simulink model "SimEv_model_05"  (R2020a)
settings: Solver=VariableStepAuto  StartTime=0.0  StopTime=10.0  RelTol=1e-3
undefined symbols (not defined in the file): m, n

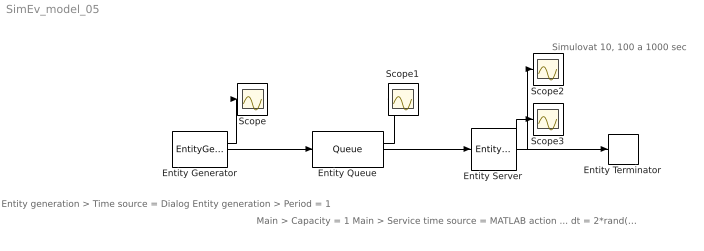
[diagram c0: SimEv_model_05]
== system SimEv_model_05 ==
  note: Simulovat 10, 100 a 1000 sec
  note: Entity generation > Time source = Dialog Entity generation > Period = 1
  note: Main > Capacity = 1 Main > Service time source = MATLAB action ... dt = 2*rand(1,1)
  Entity Generator : EntityGenerator  OutputPortMessageModes=n,m  IntergenerationTimeAction=|  NumberEntitiesDeparted=on  EntityType=Structured  EntityTypeName=Entity
      | persistent rngInit;
      | if isempty(rngInit)
      |     seed = 12345;
      |     rng(seed);
      |     rngInit = true;
      | end
      | 
      | % Pattern: Exponential distribution
      | mu = 1;
      | dt = -mu * log(1 - rand());
  Entity Queue : Queue  InputPortMessageModes=m  OutputPortMessageModes=n,m  NumberEntitiesInBlock=on
  Entity Server : EntityServer  InputPortMessageModes=m  OutputPortMessageModes=n,n,m  Capacity=1  ServiceTimeSource=MATLAB action  ServiceTimeValue=1  ServiceTimeAction=dt = 2*rand(1,1);  NumberEntitiesDeparted=on  NumberEntitiesInBlock=on
  Entity Terminator : EntityTerminator  InputPortMessageModes=m
  Scope{,1..3} (4 alike) : Scope
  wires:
  Entity Generator/1 -> Scope/1
  Entity Generator/2 -> Entity Queue/1
  Entity Queue/2 -> Entity Server/1
  Entity Server/3 -> Entity Terminator/1
  Entity Queue/1 -> Scope1/1
  Entity Server/2 -> Scope2/1
  Entity Server/1 -> Scope3/1
